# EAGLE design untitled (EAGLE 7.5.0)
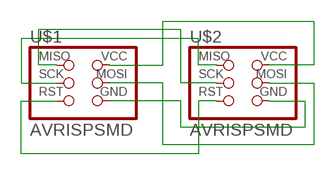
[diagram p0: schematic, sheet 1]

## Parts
U$1  AVRISPSMD  [2X03SMD]
U$2  AVRISPSMD  [2X03SMD]

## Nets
N$1: U$1.2(VCC) U$2.2(VCC)
N$2: U$1.4(MOSI) U$2.4(MOSI)
N$3: U$1.6(GND) U$2.6(GND)
N$4: U$1.5(RST) U$2.5(RST)
N$5: U$1.3(SCK) U$2.1(MISO)
N$6: U$1.1(MISO) U$2.3(SCK)

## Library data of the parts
U$1 U$2 = fab:AVRISP

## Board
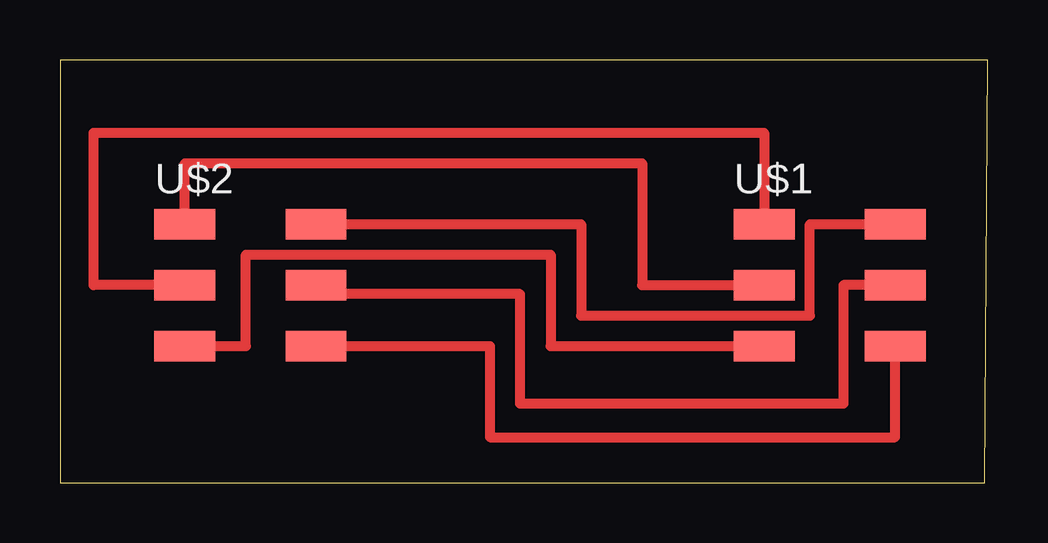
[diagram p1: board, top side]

Size 38.66 x 17.64 mm. Coordinates in mm from the lower left corner, seen from the top.
Outline: 0,0 38.53,0 38.66,17.64 0,17.64 0,0
Copper layers (1*16): Top 0.035mm / dielectric 1.5mm / Bottom 0.035mm
Design rules "default": minimum track width 10mil, minimum drill 24mil, track to track 8mil, track to pad 8mil, pad to pad 8mil, via to via 8mil, smd to smd 8mil, copper to edge 40mil, drill to drill 8mil, minimum pad ring 10mil, minimum via ring 8mil, stop-mask expansion 4mil, vias tented up to drill 0mil, thermal gap 10mil

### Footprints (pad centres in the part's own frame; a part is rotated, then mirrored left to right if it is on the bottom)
2X03SMD = smd 2.54 x 1.27: 1 -2.54,2.54; 2 2.92,2.54; 3 -2.54,0; 4 2.92,0; 5 -2.54,-2.54; 6 2.92,-2.54

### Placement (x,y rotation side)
U$1  31.88,8.26 0 top
U$2  7.75,8.26 0 top

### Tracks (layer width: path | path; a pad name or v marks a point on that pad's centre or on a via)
N$1
  Top 0.406: U$2.2 21.72,10.8 21.72,6.99 31.24,6.99 31.24,10.8 U$1.2
N$2
  Top 0.406: U$1.4 32.64,8.26 32.64,3.3 19.18,3.3 19.18,7.87 10.67,7.87 U$2.4
N$3
  Top 0.406: U$2.6 17.91,5.72 17.91,1.91 34.8,1.91 U$1.6
N$4
  Top 0.406: U$2.5 7.75,5.72 7.75,9.53 20.45,9.53 20.45,5.72 U$1.5
N$5
  Top 0.406: U$2.1 5.21,13.34 24.26,13.34 24.26,8.26 U$1.3
N$6
  Top 0.406: U$2.3 1.4,8.26 1.4,14.61 29.34,14.61 U$1.1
